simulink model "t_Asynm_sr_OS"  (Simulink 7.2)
settings: Solver=ode3  StartTime=0.0  StopTime=1  FixedStep=1e-5  MaxStep=1e-4  RelTol=1e-4  AbsTol=1e-4
libraries: simulink x1

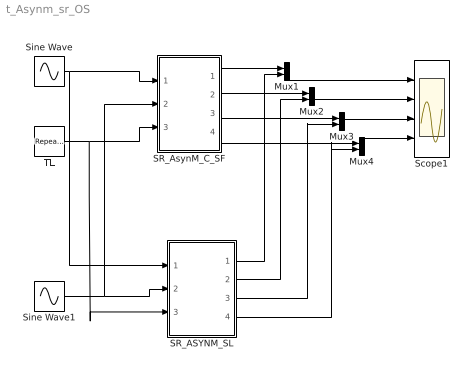
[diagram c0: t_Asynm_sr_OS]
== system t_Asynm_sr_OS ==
  Mux{1..4} (4 alike) : Mux  Inputs=2
  SR_ASYNM_SL : Subsystem  mask(SR_Asyn_Motor_SL){rs=0.087, Lls=0.8e-3, rr=0.228, Llr=0.8e-3, Lm=34.7e-3, N12=1, P=4, J=0.8, D=0.1, omm0=0}
      mask prompts: rs "Stator Resistance"; Lls "Stator Leakage Inductance"; rr "Rotor Resistance'"; Llr "Rotor Leakage Inductance'"; Lm "Magnetising Inductance"; N12 "Turns Ratio"; P "Number of Poles"; J "Moment of Inertia"; D "Damping Coefficient"; omm0 "initial ang. speed"
      mask help: Open source Slip Ring Asyn. MOTOR modeled in Simulink Blocks Input Vector u: u[0,1,2]= Three phase stator Voltages u[3,4,5]= Three phase Rotor Voltages u[6]= Load Torque Output Vector y: y[0,1,2]= Three phase stator Currents y[3,4,5]= Three phase Rotor Currents y[6]= Te y[7]= Ang. Velocity W Parameter Vector p: p[0]= Rs p[1]= Ls p[2]= Rr p[3]= Lr p[4]= LM p[5]= Turns Ratio p[6]= Number of Poles P p[7]= Moment of Inertia J p[8]= Damp. Coef. D p[9]= Initial Ang. Velocity W0 You can pause the simulation during running, change the Parameters you want and continue the Simulation
  SR_AsynM_C_SF : Subsystem  mask(SR_ASYN_MOTOR_C-SF){RS=0.087, LS=0.8e-3, RR=0.228, LR=0.8e-3, LM=34.7e-3, N12=1, P=4, J=0.8, D=0.1, W0=0}
      mask prompts: RS "Stator Resistance"; LS "Stator Leakage Inductance"; RR "Rotor Resistance"; LR "Rotor Leakage Inductance"; LM "Magnetising Inductance"; N12 "Turns ratio"; P "Number of Poles"; J "Moment of Inertia"; D "Damping Coefficient"; W0 "initial ang. speed"
      mask help: Open source Slip Ring Asyn. MOTOR modeled as Simulink C-S-Function Block Input Vector u: u[0,1,2]= Three phase stator Voltages u[3,4,5]= Three phase Rotor Voltages u[6]= Load Torque Output Vector y: y[0,1,2]= Three phase stator Currents y[3,4,5]= Three phase Rotor Currents y[6]= Te y[7]= Ang. Velocity W Parameter Vector p: p[0]= Rs p[1]= Ls p[2]= Rr p[3]= Lr p[4]= LM p[5]= Turns Ratio p[6]= Number of Poles P p[7]= Moment of Inertia J p[8]= Damp. Coef. D p[9]= Initial Ang. Velocity W0 You can pause the simulation during running, change the Parameters you want and continue the Simulation
  Scope1 : Scope  NumInputPorts=4
  Sine Wave : Sin  Amplitude=400*sqrt(2)  Frequency=50*2*pi  Phase=[0, -2*pi/3, -4*pi/3]  SampleTime=0
  Sine Wave1 : Sin  Amplitude=0  Frequency=50*2*pi  Phase=[0, -2*pi/3, -4*pi/3]  SampleTime=0
  TL : simulink/Sources/Repeating Sequence  SystemSampleTime=-1  rep_seq_t="[0      0.3     0.301      0.6    0.601     1 ]"  rep_seq_y="[0       0         1            1        -1         -1]*1000"
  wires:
  Sine Wave/1 -> SR_AsynM_C_SF/1(V1abc), SR_ASYNM_SL/1(V1abc)
  TL/1 -> SR_AsynM_C_SF/3(TL), SR_ASYNM_SL/3(Tl)
  Sine Wave1/1 -> SR_AsynM_C_SF/2(V2abc), SR_ASYNM_SL/2(V2abc)
  Mux1/1 -> Scope1/1
  SR_AsynM_C_SF/1(i1abc) -> Mux1/1
  SR_ASYNM_SL/1(I1abc) -> Mux1/2
  SR_AsynM_C_SF/2(i2abc) -> Mux2/1
  SR_ASYNM_SL/2(I2abc) -> Mux2/2
  Mux2/1 -> Scope1/2
  Mux3/1 -> Scope1/3
  SR_AsynM_C_SF/3(TE) -> Mux3/1
  SR_ASYNM_SL/3(Te) -> Mux3/2
  SR_AsynM_C_SF/4(W) -> Mux4/1
  SR_ASYNM_SL/4(w) -> Mux4/2
  Mux4/1 -> Scope1/4

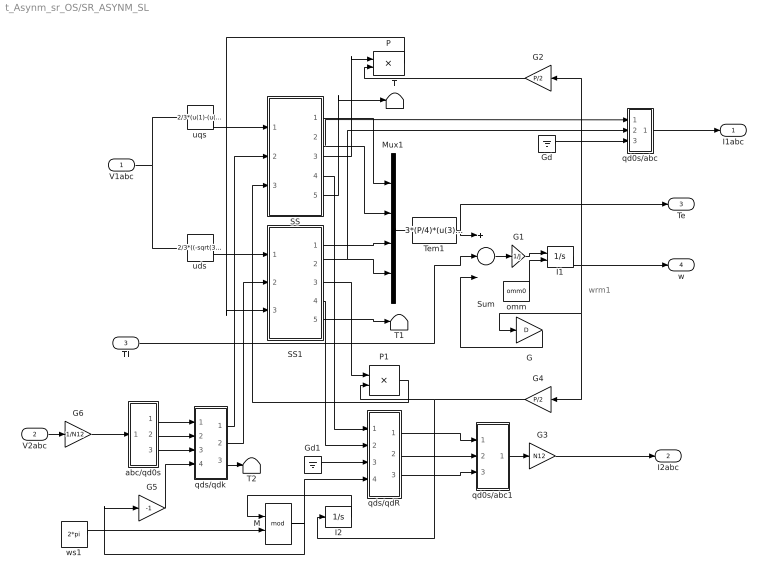
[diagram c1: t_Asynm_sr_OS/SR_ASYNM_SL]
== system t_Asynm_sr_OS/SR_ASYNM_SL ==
  note: wrm1
  V1abc : Inport
  V2abc : Inport  Port=2
  Tl : Inport  Port=3
  G : Gain  Gain=D
  G1 : Gain  Gain=1/J
  G2 : Gain  Orientation=left  Gain=P/2
  G3 : Gain  Gain=N12
  G4 : Gain  Orientation=left  Gain=P/2
  G5 : Gain  Gain=-1
  G6 : Gain  Gain=1/N12
  Gd : Ground
  Gd1 : Ground
  I1 : Integrator  InitialConditionSource=external
  I2 : Integrator
  M : Math  Operator=mod
  Mux1 : Mux
  P : Product
  P1 : Product
  SS : Subsystem
  SS1 : Subsystem
  Sum : Sum  Inputs=+--
  T : Terminator
  T1 : Terminator
  T2 : Terminator
  Tem1 : Fcn  Expr=3*(P/4)*(u(3)*u(2)-u(1)*u(4))
  abc/qd0s : Subsystem
  omm : Constant  Value=omm0
  qd0s/abc : Subsystem
  qd0s/abc1 : Subsystem
  qds/qdR : Subsystem
  qds/qdk : Subsystem
  uds : Fcn  Expr=2/3*((-sqrt(3)/2)*u(2)+(sqrt(3)/2)*u(3))
  uqs : Fcn  Expr=2/3*(u(1)-(u(2)/2)-(u(3)/2))
  ws1 : Constant  Value=2*pi
  I1abc : Outport
  I2abc : Outport  Port=2
  Te : Outport  Port=3
  w : Outport  Port=4
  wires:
  omm/1 -> I1/2
  G1/1 -> I1/1
  qds/qdk/3(0k) -> T2/1
  SS1/5(psidm) -> T1/1
  SS/5(psiqm) -> T/1
  qd0s/abc/1(a) -> I1abc/1
  qd0s/abc1/1(a) -> G3/1
  qds/qdR/1(qk) -> qd0s/abc1/1(q)
  qds/qdR/2(dk) -> qd0s/abc1/2(d)
  qds/qdR/3(0k) -> qd0s/abc1/3(0)
  Mux1/1 -> Tem1/1
  Sum/1 -> G1/1
  G2/1 -> P/2
  G4/1 -> P1/2, I2/1
  uqs/1 -> SS/1(uqs)
  uds/1 -> SS1/1(uds)
  P1/1 -> SS/3(wr*ps)
  P/1 -> SS1/3(wr*ps)
  I1/1 -> G/1, G4/1, G2/1, w/1
  G/1 -> Sum/3
  SS/2(iqs) -> Mux1/2, qd0s/abc/1(q)
  Tem1/1 -> Sum/1, Te/1
  Tl/1 -> Sum/2
  SS/1(psiqs) -> Mux1/1
  SS/3(psiqr) -> P/1
  SS1/3(psidr) -> P1/1
  SS1/2(ids) -> Mux1/4, qd0s/abc/2(d)
  SS1/1(psids) -> Mux1/3
  Gd/1 -> qd0s/abc/3(0)
  SS/4(iqr) -> qds/qdR/1(qs)
  SS1/4(idr) -> qds/qdR/2(ds)
  Gd1/1 -> qds/qdR/3(0s)
  I2/1 -> M/1
  ws1/1 -> M/2
  M/1 -> G5/1, qds/qdR/4(th)
  abc/qd0s/2(d) -> qds/qdk/2(ds)
  abc/qd0s/1(q) -> qds/qdk/1(qs)
  abc/qd0s/3(0) -> qds/qdk/3(0s)
  G5/1 -> qds/qdk/4(th)
  qds/qdk/1(qk) -> SS/2(uqr)
  qds/qdk/2(dk) -> SS1/2(udr)
  V1abc/1 -> uqs/1, uds/1
  V2abc/1 -> G6/1
  G3/1 -> I2abc/1
  G6/1 -> abc/qd0s/1(a)

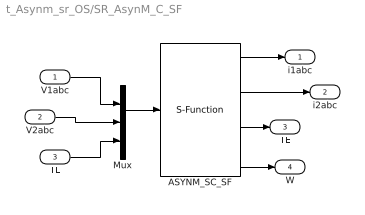
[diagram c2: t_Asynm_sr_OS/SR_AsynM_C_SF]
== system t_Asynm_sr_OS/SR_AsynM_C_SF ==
  V1abc : Inport  OutDataType=sfix(16)  OutScaling=2^0
  V2abc : Inport  Port=2  OutDataType=sfix(16)  OutScaling=2^0
  TL : Inport  Port=3  OutDataType=sfix(16)  OutScaling=2^0
  ASYNM_SC_SF : S-Function  FunctionName=s_Asynm_sr_OS  Parameters="[RS LS RR LR LM  N12  P J D W0]"  EnableBusSupport=off
  Mux : Mux  Inputs="[3  3  1]"
  i1abc : Outport  OutDataType=sfix(16)  OutScaling=2^0
  i2abc : Outport  Port=2  OutDataType=sfix(16)  OutScaling=2^0
  TE : Outport  Port=3  OutDataType=sfix(16)  OutScaling=2^0
  W : Outport  Port=4  OutDataType=sfix(16)  OutScaling=2^0
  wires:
  ASYNM_SC_SF/4 -> W/1
  ASYNM_SC_SF/1 -> i1abc/1
  ASYNM_SC_SF/3 -> TE/1
  ASYNM_SC_SF/2 -> i2abc/1
  V1abc/1 -> Mux/1
  Mux/1 -> ASYNM_SC_SF/1
  TL/1 -> Mux/3
  V2abc/1 -> Mux/2

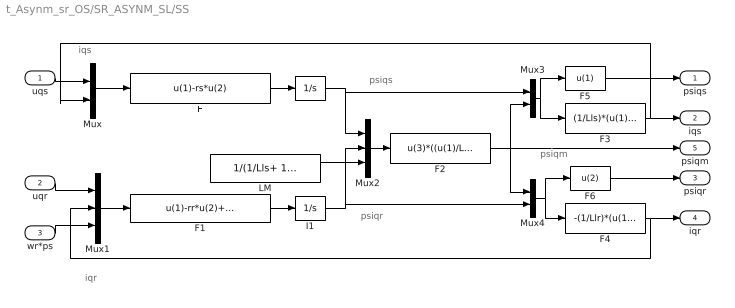
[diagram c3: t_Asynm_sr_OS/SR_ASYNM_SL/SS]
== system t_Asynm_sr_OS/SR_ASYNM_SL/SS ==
  note: psiqs
  note: psiqm
  note: psiqr
  note: iqr
  note: iqs
  uqs : Inport
  uqr : Inport  Port=2
  wr*ps : Inport  Port=3
  F : Fcn  Expr=u(1)-rs*u(2)
  F1 : Fcn  Expr=u(1)-rr*u(2)+u(3)
  F2 : Fcn  Expr=u(3)*((u(1)/Lls)+(u(2)/Llr))
  F3 : Fcn  Expr=(1/Lls)*(u(1)-u(2))
  F4 : Fcn  Expr=-(1/Llr)*(u(1)-u(2))
  F5 : Fcn  Expr=u(1)
  F6 : Fcn  Expr=u(2)
  I : Integrator
  I1 : Integrator
  LM : Constant  Value=1/(1/Lls+ 1/Llr+ 1/Lm)
  Mux : Mux  Inputs=2
  Mux1 : Mux  Inputs=3
  Mux2 : Mux  Inputs=3
  Mux3 : Mux  Inputs=2
  Mux4 : Mux  Inputs=2
  psiqs : Outport
  iqs : Outport  Port=2
  psiqr : Outport  Port=3
  iqr : Outport  Port=4
  psiqm : Outport  Port=5
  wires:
  Mux/1 -> F/1
  F/1 -> I/1
  Mux1/1 -> F1/1
  Mux2/1 -> F2/1
  F2/1 -> Mux3/2, Mux4/1, psiqm/1
  I/1 -> Mux2/1, Mux3/1
  I1/1 -> Mux4/2, Mux2/2
  uqs/1 -> Mux/1
  Mux3/1 -> F3/1, F5/1
  F5/1 -> psiqs/1
  Mux4/1 -> F4/1, F6/1
  F6/1 -> psiqr/1
  F1/1 -> I1/1
  uqr/1 -> Mux1/1
  F3/1 -> iqs/1, Mux/2
  wr*ps/1 -> Mux1/3
  F4/1 -> iqr/1, Mux1/2
  LM/1 -> Mux2/3

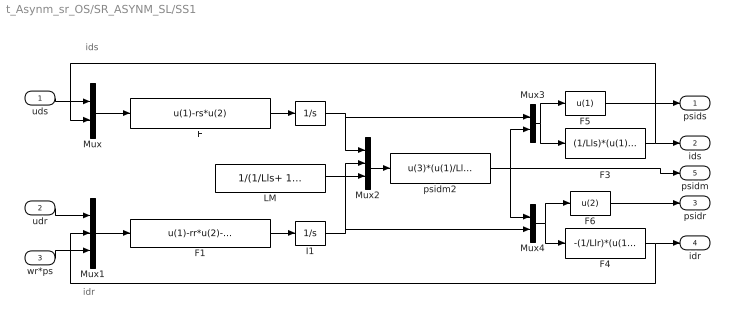
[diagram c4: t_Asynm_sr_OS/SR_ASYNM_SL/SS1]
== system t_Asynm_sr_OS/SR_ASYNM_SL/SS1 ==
  note: ids
  note: idr
  uds : Inport
  udr : Inport  Port=2
  wr*ps : Inport  Port=3
  F : Fcn  Expr=u(1)-rs*u(2)
  F1 : Fcn  Expr=u(1)-rr*u(2)-u(3)
  F3 : Fcn  Expr=(1/Lls)*(u(1)-u(2))
  F4 : Fcn  Expr=-(1/Llr)*(u(1)-u(2))
  F5 : Fcn  Expr=u(1)
  F6 : Fcn  Expr=u(2)
  I : Integrator
  I1 : Integrator
  LM : Constant  Value=1/(1/Lls+ 1/Llr+ 1/Lm)
  Mux : Mux  Inputs=2
  Mux1 : Mux  Inputs=3
  Mux2 : Mux  Inputs=3
  Mux3 : Mux  Inputs=2
  Mux4 : Mux  Inputs=2
  psidm2 : Fcn  Expr=u(3)*(u(1)/Lls+u(2)/Llr)
  psids : Outport
  ids : Outport  Port=2
  psidr : Outport  Port=3
  idr : Outport  Port=4
  psidm : Outport  Port=5
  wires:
  F6/1 -> psidr/1
  Mux4/1 -> F6/1, F4/1
  F5/1 -> psids/1
  Mux3/1 -> F5/1, F3/1
  uds/1 -> Mux/1
  I1/1 -> Mux4/2, Mux2/2
  I/1 -> Mux3/1, Mux2/1
  Mux2/1 -> psidm2/1
  Mux1/1 -> F1/1
  F/1 -> I/1
  Mux/1 -> F/1
  F1/1 -> I1/1
  wr*ps/1 -> Mux1/3
  udr/1 -> Mux1/1
  F3/1 -> ids/1, Mux/2
  F4/1 -> idr/1, Mux1/2
  LM/1 -> Mux2/3
  psidm2/1 -> Mux3/2, Mux4/1, psidm/1

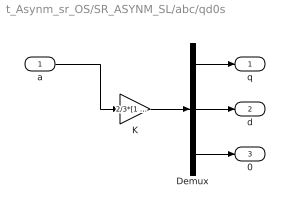
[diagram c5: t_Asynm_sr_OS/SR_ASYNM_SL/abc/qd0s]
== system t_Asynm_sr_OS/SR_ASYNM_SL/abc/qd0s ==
  a : Inport
  Demux : Demux  Outputs=3
  K : Gain  Gain="2/3*[1   -.5   -.5;  0   -sqrt(3)/2   sqrt(3)/2;  .5    .5    .5]"  Multiplication=Matrix(K*u)
  q : Outport
  d : Outport  Port=2
  0 : Outport  Port=3
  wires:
  K/1 -> Demux/1
  a/1 -> K/1
  Demux/1 -> q/1
  Demux/2 -> d/1
  Demux/3 -> 0/1

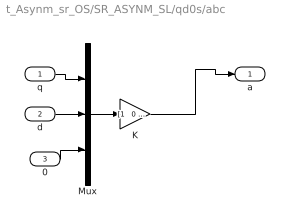
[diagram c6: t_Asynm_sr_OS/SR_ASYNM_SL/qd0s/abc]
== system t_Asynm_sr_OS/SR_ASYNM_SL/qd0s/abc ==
  q : Inport
  d : Inport  Port=2
  0 : Inport  Port=3
  K : Gain  Gain="[1   0  1;  -.5   -sqrt(3)/2   1;  -.5    sqrt(3)/2  1]"  Multiplication=Matrix(K*u)
  Mux : Mux  Inputs=3
  a : Outport
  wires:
  q/1 -> Mux/1
  0/1 -> Mux/3
  Mux/1 -> K/1
  K/1 -> a/1
  d/1 -> Mux/2

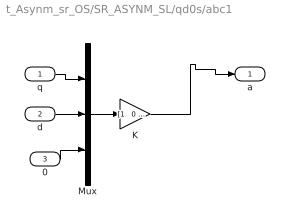
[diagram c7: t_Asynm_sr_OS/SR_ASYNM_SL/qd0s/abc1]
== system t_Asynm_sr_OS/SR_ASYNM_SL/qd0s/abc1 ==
  q : Inport
  d : Inport  Port=2
  0 : Inport  Port=3
  K : Gain  Gain="[1   0  1;  -.5   -sqrt(3)/2   1;  -.5    sqrt(3)/2  1]"  Multiplication=Matrix(K*u)
  Mux : Mux  Inputs=3
  a : Outport
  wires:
  d/1 -> Mux/2
  K/1 -> a/1
  Mux/1 -> K/1
  0/1 -> Mux/3
  q/1 -> Mux/1

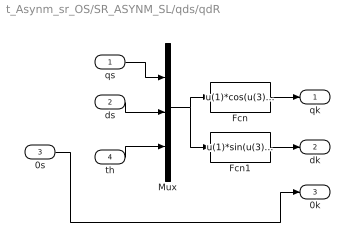
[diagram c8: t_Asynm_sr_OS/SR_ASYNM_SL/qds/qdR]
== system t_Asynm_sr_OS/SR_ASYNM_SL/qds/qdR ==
  qs : Inport  OutDataType=sfix(16)  OutScaling=2^0
  ds : Inport  Port=2  OutDataType=sfix(16)  OutScaling=2^0
  0s : Inport  Port=3  OutDataType=sfix(16)  OutScaling=2^0
  th : Inport  Port=4  OutDataType=sfix(16)  OutScaling=2^0
  Fcn : Fcn  Expr=u(1)*cos(u(3)) - u(2)*sin(u(3))
  Fcn1 : Fcn  Expr=u(1)*sin(u(3)) + u(2)*cos(u(3))
  Mux : Mux  Inputs=3
  qk : Outport
  dk : Outport  Port=2
  0k : Outport  Port=3
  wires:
  Fcn1/1 -> dk/1
  Fcn/1 -> qk/1
  Mux/1 -> Fcn1/1, Fcn/1
  ds/1 -> Mux/2
  qs/1 -> Mux/1
  0s/1 -> 0k/1
  th/1 -> Mux/3

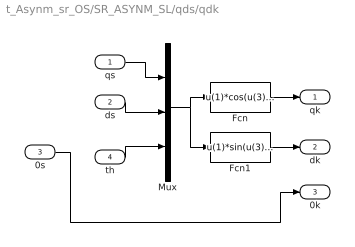
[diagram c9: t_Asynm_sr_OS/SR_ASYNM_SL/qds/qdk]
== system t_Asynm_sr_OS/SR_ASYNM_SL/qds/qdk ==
  qs : Inport  OutDataType=sfix(16)  OutScaling=2^0
  ds : Inport  Port=2  OutDataType=sfix(16)  OutScaling=2^0
  0s : Inport  Port=3  OutDataType=sfix(16)  OutScaling=2^0
  th : Inport  Port=4  OutDataType=sfix(16)  OutScaling=2^0
  Fcn : Fcn  Expr=u(1)*cos(u(3)) - u(2)*sin(u(3))
  Fcn1 : Fcn  Expr=u(1)*sin(u(3)) + u(2)*cos(u(3))
  Mux : Mux  Inputs=3
  qk : Outport
  dk : Outport  Port=2
  0k : Outport  Port=3
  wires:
  Fcn1/1 -> dk/1
  Fcn/1 -> qk/1
  Mux/1 -> Fcn1/1, Fcn/1
  ds/1 -> Mux/2
  qs/1 -> Mux/1
  0s/1 -> 0k/1
  th/1 -> Mux/3
